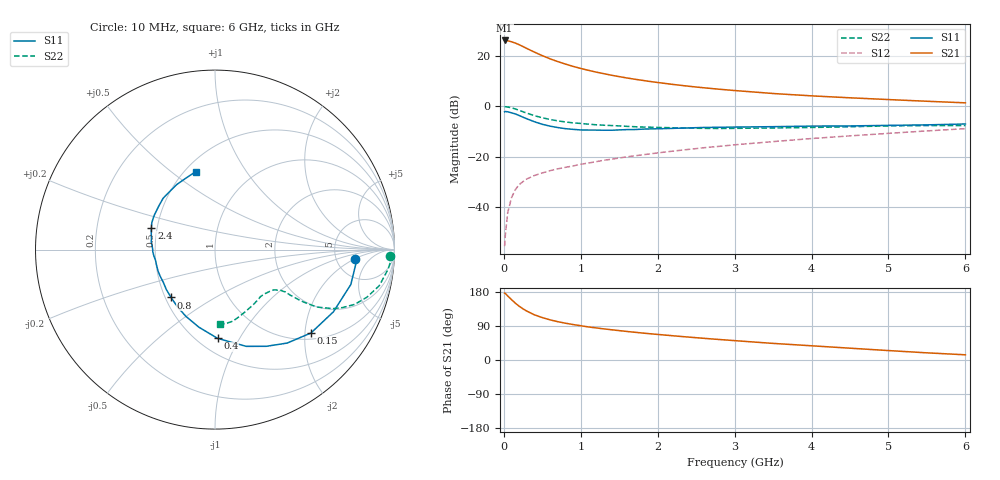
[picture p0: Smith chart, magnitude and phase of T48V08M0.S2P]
! Infineon Technologies  Discrete & RF Semiconductors
! BFR182T
! Si NPN RF Bipolar Junction Transistor in SC75
! VCE = 8 V  IC = 8 mA
! Common Emitter S-Parameters:  October  1999
# GHz  S  MA  R  50
!  f  S11  S21  S12  S22
! GHz  MAG  ANG  MAG  ANG  MAG  ANG  MAG  ANG
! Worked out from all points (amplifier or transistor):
!   36 points, 10 MHz to 6 GHz, reference 50 ohm
!   highest |S21| = 26.1 dB at 10 MHz (marker M1)
!   |S21| within 3 dB of that: start of sweep to 287.2 MHz
!   unconditionally stable (mu >= 1): 1.222 GHz to 4.02 GHz
!   at 250 MHz: K = 0.37, MSG = 26.7 dB, |S12| = -29.8 dB
!   at 1.4 GHz: K = 1.04, MAG = 15.5 dB, |S12| = -20.9 dB
!   at 6 GHz: K = 0.86, MSG = 5.1 dB, |S12| = -8.8 dB
!   lowest NFmin = 1.40 dB at 450 MHz
!   S11 on the Smith chart (normalised r, x): 10 MHz: 7.57, -2.07; 150 MHz: 1.15, -2.15; 400 MHz: 0.62, -0.81; 800 MHz: 0.54, -0.33; 2.4 GHz: 0.47, +0.13; 6 GHz: 0.57, +0.62
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0.01  0.7813 -3.9  20.23 176.5  0.0017 93.4  0.9757 -2.0
0.02  0.7916 -4.4  20.22 175.5  0.0029 96.6  0.9857 -2.6
0.05  0.7814 -14.4  19.96 169.0  0.0078 84.5  0.9705 -6.5
0.1  0.7453 -27.7  19.05 159.3  0.0156 79.2  0.9371 -12.4
0.15  0.7082 -41.0  17.95 149.9  0.0225 71.2  0.887 -17.4
0.2  0.6581 -52.3  16.66 141.8  0.0283 68.3  0.8362 -21.4
0.25  0.6097 -62.1  15.28 134.9  0.0324 63.3  0.7815 -24.4
0.3  0.5665 -72.1  14.01 128.9  0.0366 61.8  0.7347 -26.6
0.4  0.4948 -88.3  11.84 119.0  0.0429 58.5  0.6523 -29.4
0.5  0.4416 -101.7  10.12 111.9  0.0479 57.3  0.5953 -30.3
0.6  0.4059 -113.5  8.765 106.0  0.0532 56.8  0.551 -30.9
0.7  0.3809 -123.5  7.729 101.2  0.0578 57.5  0.5168 -31.0
0.8  0.3619 -132.5  6.896 97.1  0.062 58.1  0.4921 -31.2
1.1  0.3395 -154.5  5.179 87.2  0.0756 60.0  0.4444 -31.5
1.4  0.3368 -169.8  4.14 79.8  0.0898 61.6  0.4172 -32.9
1.6  0.3469 -178.0  3.654 75.3  0.1001 62.3  0.4021 -33.9
2.2  0.367 165.4  2.719 63.9  0.13 63.5  0.3771 -39.4
2.4  0.3742 161.2  2.509 60.5  0.1405 63.8  0.3703 -41.7
3.5  0.3963 142.2  1.8 43.8  0.2006 61.7  0.3736 -55.1
4.5  0.4099 128.5  1.479 31.2  0.2604 58.0  0.395 -69.1
5.5  0.4303 111.8  1.263 18.9  0.3266 53.1  0.4159 -81.1
6  0.4479 103.8  1.175 13.7  0.3618 49.8  0.4164 -86.0
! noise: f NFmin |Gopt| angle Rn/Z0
0.45  1.4  0.26  41  0.29
0.9  1.5  0.25  83  0.23
1.8  2  0.21  162  0.2
